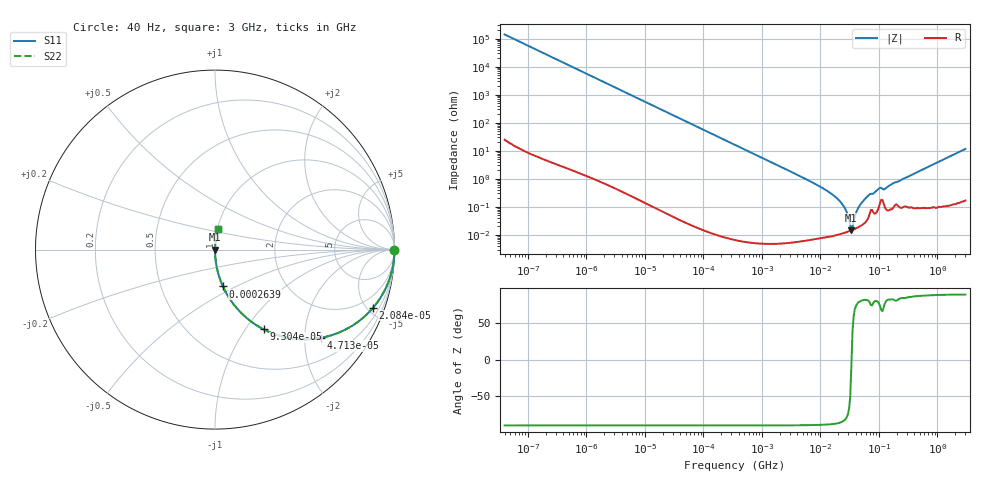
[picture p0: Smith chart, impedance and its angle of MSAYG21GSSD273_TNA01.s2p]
! MSAYG21GSSD273_TNA01  S-PARAMETER MODEL  ( General Type )
! Model Generated by TAIYO YUDEN Corporation (http://www.ty-top.com)
! Version 2.0
! TAIYO YUDEN Control No. 031016
! Copyright(c) 2003 TAIYO YUDEN CO.,LTD. All Rights Reserved.
! Product Description (link to TY-COMPAS)
! https://ds.yuden.co.jp/TYCOMPAS/or/detail?pn=MSAYG21GSSD273KTNA01&u=M
! Products Name : Multilayer Ceramic Capacitors
! Characteristics :
!  Capacitance : 0.027 uF , Rated Voltage : 35V
!  Case Size : 2.0 x 1.25 / 0.079 x 0.049 [mm/inch] , Thickness : 1.25 / 0.049 [mm/inch]
!  (Conditions: Temperature = 25 degC , DC Bias Current/Voltage = 0A / 0V)
! External Node Assignments :
!  1  o---| |---o  2
! GND o---------o GND
! Frequency Range : 40Hz  -  3GHz  [ 401 STEP ]
# MHz S RI R 50
! Freq[MHz].  S11 Real  S11 Imag  S21 Real  S21 Imag  S12 Real  S12 Imag  S22 Real  S22 Imag
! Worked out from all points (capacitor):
!   401 points, 40 Hz to 3 GHz, reference 50 ohm
!   read as one part in series: C = 28 nF near 44 Hz
!   lowest |Z| = 14.4 mohm at 33.73 MHz (marker M1)
!   series resonance near 34 MHz, so ESL is about 780 pH
!   S11 on the Smith chart (normalised r, x): 40 Hz: open; 20.84 kHz: 1.00, -5.44; 47.13 kHz: 1.00, -2.41; 93.03 kHz: 1.00, -1.22; 263.9 kHz: 1.00, -0.43; 3 GHz: 1.00, +0.23
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4e-05  1 -0.000705  6.2e-07 0.000705  6.2e-07 0.000705  1 -0.000705
0.000834  0.9998 -0.0147  0.000219 0.0147  0.000219 0.0147  0.9998 -0.0147
0.005113  0.9919 -0.0894  0.00808 0.0894  0.00808 0.0894  0.9919 -0.0894
0.017386  0.9141 -0.2801  0.0859 0.2801  0.0859 0.2801  0.9141 -0.2801
0.020843  0.8811 -0.3236  0.1189 0.3236  0.1189 0.3236  0.8811 -0.3236
0.047134  0.5917 -0.4914  0.4083 0.4914  0.4083 0.4914  0.5917 -0.4914
0.093035  0.2712 -0.4444  0.7288 0.4444  0.7288 0.4444  0.2712 -0.4444
0.263915  0.0442 -0.2055  0.9558 0.2055  0.9558 0.2055  0.0442 -0.2055
0.362475  0.024 -0.1528  0.976 0.1528  0.976 0.1528  0.024 -0.1528
7.222098  0.000124 -0.0075  0.9999 0.0075  0.9999 0.0075  0.000124 -0.0075
13.62356  9.75e-05 -0.00349  0.9999 0.00349  0.9999 0.00349  9.75e-05 -0.00349
20.48705  0.000106 -0.00176  0.9999 0.00176  0.9999 0.00176  0.000106 -0.00176
25.69909  0.000119 -0.000949  0.9999 0.000949  0.9999 0.000949  0.000119 -0.000949
32.2371  0.00014 -0.000175  0.9999 0.000175  0.9999 0.000175  0.00014 -0.000175
33.73212  0.000142 -2.44e-05  0.9999 2.44e-05  0.9999 2.44e-05  0.000142 -2.44e-05
36.93337  0.000159 0.000265  0.9998 -0.000265  0.9998 -0.000265  0.000159 0.000265
44.27611  0.000186 0.000891  0.9998 -0.000891  0.9998 -0.000891  0.000186 0.000891
60.81113  0.000312 0.00213  0.9997 -0.00213  0.9997 -0.00213  0.000312 0.00213
100.1261  0.00104 0.00438  0.999 -0.00438  0.999 -0.00438  0.00104 0.00438
125.5988  0.00102 0.00418  0.999 -0.00418  0.999 -0.00418  0.00102 0.00418
150.5692  0.000806 0.00569  0.9992 -0.00569  0.9992 -0.00569  0.000806 0.00569
3000  0.015 0.1145  0.985 -0.1145  0.985 -0.1145  0.015 0.1145
